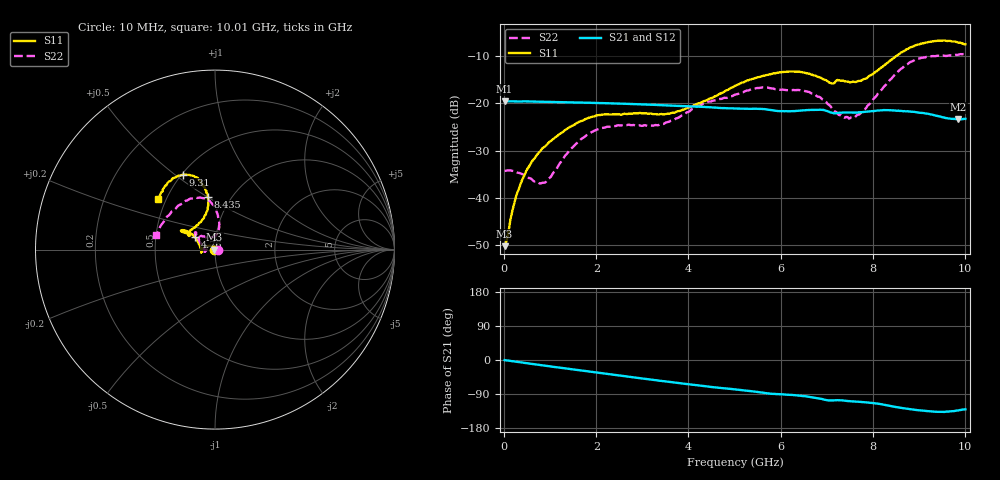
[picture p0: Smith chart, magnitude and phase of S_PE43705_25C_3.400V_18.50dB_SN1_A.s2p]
! Device ID: PE43705
! Serial: 1
! Insertion: A
! Impedance: 50 ohm
! Temp: 25C
! VDD: 3.400V
! Attenuation Step: 18.50dB
#  Hz  S  RI  R  50
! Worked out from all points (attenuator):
!   401 points, 10 MHz to 10.01 GHz, reference 50 ohm
!   highest |S21| = -19.54 dB at 10 MHz (marker M1); lowest = -23.4 dB at 9.86 GHz (marker M2)
!   lowest |S11| = -50.2 dB at 10 MHz (marker M3), VSWR 1.01, Z = 49.7 + j0.0315 ohm
!   |S11| at or under -10 dB: start of sweep to 8.513 GHz
!   |S22| runs from -37.0 to -9.5 dB; largest |S21 - S12| = 0.0011
!   S11 on the Smith chart (normalised r, x): 10 MHz: 0.99, +0.00; 4.76 GHz: 0.79, +0.11; 8.435 GHz: 0.78, +0.50; 9.31 GHz: 0.51, +0.54; 10.01 GHz: 0.45, +0.31
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1e7  -0.00308 0.000317  0.1054 -0.000419  0.1055 -0.000403  0.0193 0.000269
2.6e8  -0.00459 0.00938  0.1044 -0.00835  0.1043 -0.00827  0.0175 0.00691
5.6e8  -0.0128 0.0184  0.1028 -0.0174  0.1029 -0.0173  0.00974 0.0129
9.1e8  -0.0286 0.0215  0.1 -0.0276  0.1 -0.0275  -0.00573 0.0137
1.685e9  -0.0648 0.00777  0.0898 -0.0477  0.0899 -0.0477  -0.0424 8.3e-05
2.26e9  -0.0757 -0.0103  0.0797 -0.0606  0.0798 -0.0604  -0.0553 -0.0121
3.36e9  -0.0759 -0.00698  0.0557 -0.078  0.0558 -0.078  -0.059 0.0023
3.86e9  -0.083 0.0173  0.044 -0.0825  0.0441 -0.0824  -0.0708 0.0227
4.76e9  -0.1113 0.07  0.0239 -0.0858  0.0241 -0.0857  -0.0927 0.0659
5.01e9  -0.1272 0.0848  0.0189 -0.0861  0.019 -0.0862  -0.0986 0.0744
5.535e9  -0.1591 0.1024  0.00782 -0.0869  0.00787 -0.0869  -0.1122 0.0922
5.985e9  -0.183 0.1086  -0.000472 -0.0827  -0.000124 -0.0827  -0.1052 0.0907
6.685e9  -0.1758 0.0954  -0.0127 -0.0841  -0.0128 -0.0844  -0.0981 0.0798
7.11e9  -0.1412 0.0806  -0.0229 -0.0764  -0.0229 -0.0765  -0.0545 0.0702
7.535e9  -0.1069 0.1286  -0.0258 -0.0754  -0.0259 -0.0754  -0.00949 0.0707
7.785e9  -0.0741 0.162  -0.0291 -0.0756  -0.0286 -0.0755  0.00791 0.0838
8.36e9  -0.0363 0.2763  -0.0431 -0.0727  -0.0432 -0.0729  0.0199 0.1728
8.435e9  -0.0388 0.2936  -0.0452 -0.0711  -0.0454 -0.0714  0.0166 0.1891
8.86e9  -0.0896 0.3869  -0.053 -0.0618  -0.0523 -0.0624  -0.042 0.2751
9.31e9  -0.1765 0.4172  -0.0543 -0.0522  -0.0541 -0.052  -0.1443 0.2807
9.86e9  -0.2913 0.3252  -0.0461 -0.0493  -0.0461 -0.0493  -0.2906 0.1489
1.001e10  -0.3155 0.2792  -0.044 -0.0525  -0.0449 -0.0526  -0.326 0.084
